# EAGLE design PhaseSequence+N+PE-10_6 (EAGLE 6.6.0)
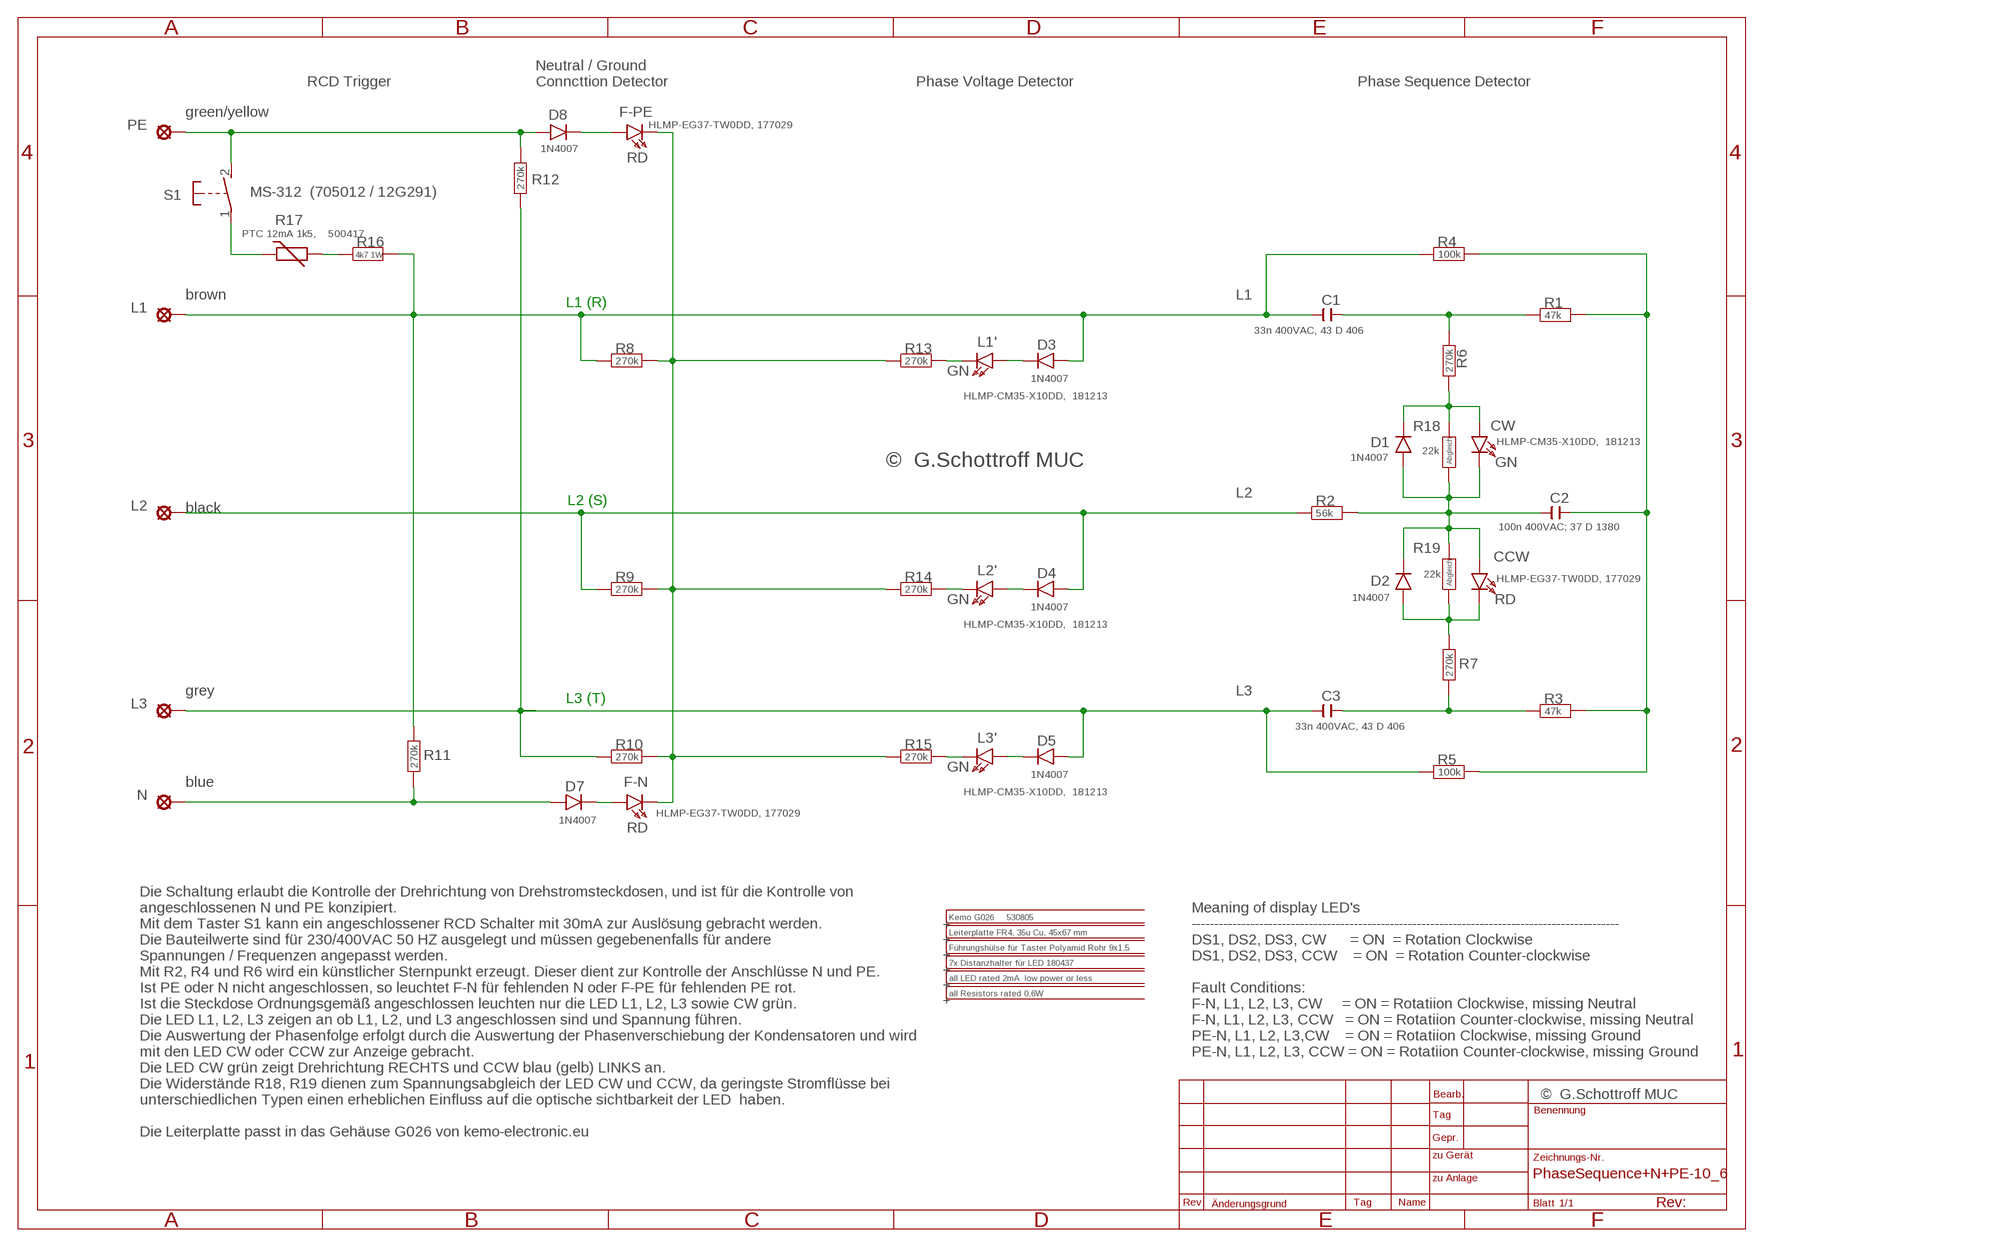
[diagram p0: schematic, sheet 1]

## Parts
C1  33n 400VAC, 43 D 406  C-EU150-064X183  [C150-064X183]
C2  100n 400VAC; 37 D 1380  C-EU150-084X183  [C150-084X183]
C3  33n 400VAC, 43 D 406  C-EU150-064X183  [C150-064X183]
CCW  HLMP-EG37-TW0DD, 177029  LED5MM  [LED5MM]
CW  HLMP-CM35-X10DD, 181213  LED5MM  [LED5MM]
D1  1N4007  1N4004  [DO41-10]
D2  1N4007  1N4004  [DO41-10]
D3  1N4007  1N4004  [DO41-10]
D4  1N4007  1N4004  [DO41-10]
D5  1N4007  1N4004  [DO41-10]
D7  1N4007  1N4004  [DO41-10]
D8  1N4007  1N4004  [DO41-10]
ENCLOSURE-1  Kemo G026 530805  KEMO-G025  [KEMO-G025]
F-N  HLMP-EG37-TW0DD, 177029  LED5MM  [LED5MM]
F-PE  HLMP-EG37-TW0DD, 177029  LED5MM  [LED5MM]
INFO1  Führungshülse für Taster Polyamid Rohr 9x1.5  INFO  [INFO]
INFO2  7x Distanzhalter für LED 180437  INFO  [INFO]
INFO3  all LED rated 2mA low power or less  INFO  [INFO]
INFO4  all Resistors rated 0,6W  INFO  [INFO]
L1  SE13  [SE13]
L1'  HLMP-CM35-X10DD, 181213  LED5MM  [LED5MM]
L2  SE13  [SE13]
L2'  HLMP-CM35-X10DD, 181213  LED5MM  [LED5MM]
L3  SE13  [SE13]
L3'  HLMP-CM35-X10DD, 181213  LED5MM  [LED5MM]
N  SE13  [SE13]
PCB  Leiterplatte FR4, 35u Cu, 45x67 mm  INFO  [INFO]
PE  SE13  [SE13]
R1  47k  R-EU_0207/10  [0207/10]
R2  56k  R-EU_0207/10  [0207/10]
R3  47k  R-EU_0207/10  [0207/10]
R4  100k  R-EU_0207/10  [0207/10]
R5  100k  R-EU_0207/10  [0207/10]
R6  270k  R-EU_0207/10  [0207/10]
R7  270k  R-EU_0207/10  [0207/10]
R8  270k  R-EU_0207/10  [0207/10]
R9  270k  R-EU_0207/10  [0207/10]
R10  270k  R-EU_0207/10  [0207/10]
R11  270k  R-EU_0207/10  [0207/10]
R12  270k  R-EU_0207/10  [0207/10]
R13  270k  R-EU_0207/10  [0207/10]
R14  270k  R-EU_0207/10  [0207/10]
R15  270k  R-EU_0207/10  [0207/10]
R16  4k7 1W  R-EU_0817/22  [P0817/22]
R17  PTC 12mA 1k5, 500417  THERMISTOR-5  [R-5]
R18  22k  R-EU_R1206  [1206]
R19  22k  R-EU_R1206  [1206]
S1  MS-312 (705012 / 12G291)  MS-312  [MS-312]

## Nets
L1: C1.2 D3.A L1.MP R4.1 R8.1 R11.2 R16.2
L2: D4.A L2.MP R2.1 R9.1
L3: C3.2 D5.A L3.MP R5.1 R10.1 R12.2
N$1: C3.1 R3.1 R7.1
N$2: C2.2 CCW.A CW.K(C) D1.A D2.C R2.2 R18.1 R19.2
N$3: C1.1 R1.1 R6.1
N$4: C2.1 R1.2 R3.2 R4.2 R5.2
N$5: CCW.K(C) D2.A R7.2 R19.1
N$6: CW.A D1.C R6.2 R18.2
N$7: F-N.K(C) F-PE.K(C) R8.2 R9.2 R10.2 R13.1 R14.1 R15.1
N$8: D7.A N.MP R11.1
N$9: L1'.K(C) R13.2
N$10: L2'.K(C) R14.2
N$11: D7.C F-N.A
N$12: D8.A PE.MP R12.1 S1.2(S)
N$13: D8.C F-PE.A
N$14: L3'.K(C) R15.2
N$15: R17.1 S1.1(P)
N$16: D3.C L1'.A
N$17: R16.1 R17.2
N$18: D4.C L2'.A
N$19: D5.C L3'.A

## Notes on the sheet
- RCD Trigger
- Neutral / Ground 
  Conncttion Detector
- Phase Voltage Detector | Phase Sequence Detector
- green/yellow
- RD
- brown
- L1 (R)
- GN
- Abgleich
- ©  G.Schottroff MUC | GN
- L2 (S)
- black
- Abgleich
- GN | RD
- grey
- L3 (T)
- GN
- blue
- RD
- Meaning of display LED's
  -----------------------------------------------------------------------------------------------
  DS1, DS2, DS3, CW      = ON  = Rotation Clockwise
  DS1, DS2, DS3, CCW    = ON  = Rotation Counter-clockwise
  
  Fault Conditions:
  F-N, L1, L2, L3, CW     = ON = Rotatiion Clockwise, missing Neutral
  F-N, L1, L2, L3, CCW   = ON = Rotatiion Counter-clockwise, missing Neutral
  PE-N, L1, L2, L3,CW    = ON = Rotatiion Clockwise, missing Ground
  PE-N, L1, L2, L3, CCW = ON = Rotatiion Counter-clockwise, missing Ground
- ©  G.Schottroff MUC
- Die Schaltung erlaubt die Kontrolle der Drehrichtung von Drehstromsteckdosen, und ist für die Kontrolle von 
  angeschlossenen N und PE konzipiert. 
  Mit dem Taster S1 kann ein angeschlossener RCD Schalter mit 30mA zur Auslösung gebracht werden.
  Die Bauteilwerte sind für 230/400VAC 50 HZ ausgelegt und müssen gegebenenfalls für andere 
  Spannungen / Frequenzen angepasst werden.
  Mit R2, R4 und R6 wird ein künstlicher Sternpunkt erzeugt. Dieser dient zur Kontrolle der Anschlüsse N und PE. 
  Ist PE oder N nicht angeschlossen, so leuchtet F-N für fehlenden N oder F-PE für fehlenden PE rot.
  Ist die Steckdose Ordnungsgemäß angeschlossen leuchten nur die LED L1, L2, L3 sowie CW grün.
  Die LED L1, L2, L3 zeigen an ob L1, L2, und L3 angeschlossen sind und Spannung führen.
  Die Auswertung der Phasenfolge erfolgt durch die Auswertung der Phasenverschiebung der Kondensatoren und wird 
  mit den LED CW oder CCW zur Anzeige gebracht.
  Die LED CW grün zeigt Drehrichtung RECHTS und CCW blau (gelb) LINKS an.
  Die Widerstände R18, R19 dienen zum Spannungsabgleich der LED CW und CCW, da geringste Stromflüsse bei 
  unterschiedlichen Typen einen erheblichen Einfluss auf die optische sichtbarkeit der LED  haben.
  
  Die Leiterplatte passt in das Gehäuse G026 von kemo-electronic.eu

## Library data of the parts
C1-C3 = rcl:C-EU: CAPACITOR, European symbol
CCW CW F-N F-PE L1' L2' L3' = led:LED: LED
D1-D5 D7 D8 = diode:1N4004: DIODE
ENCLOSURE-1 = Enclosures-DIN-Rail+more:KEMO-G025
INFO1-INFO4 PCB = frames:INFO
L1-L3 N PE = solpad:SE13: SOLDER PAD
R1-R16 R18 R19 = rcl:R-EU_: RESISTOR, European symbol
R17 = varistor:THERMISTOR: THERMISTOR
S1 = switch-misc:MS-312

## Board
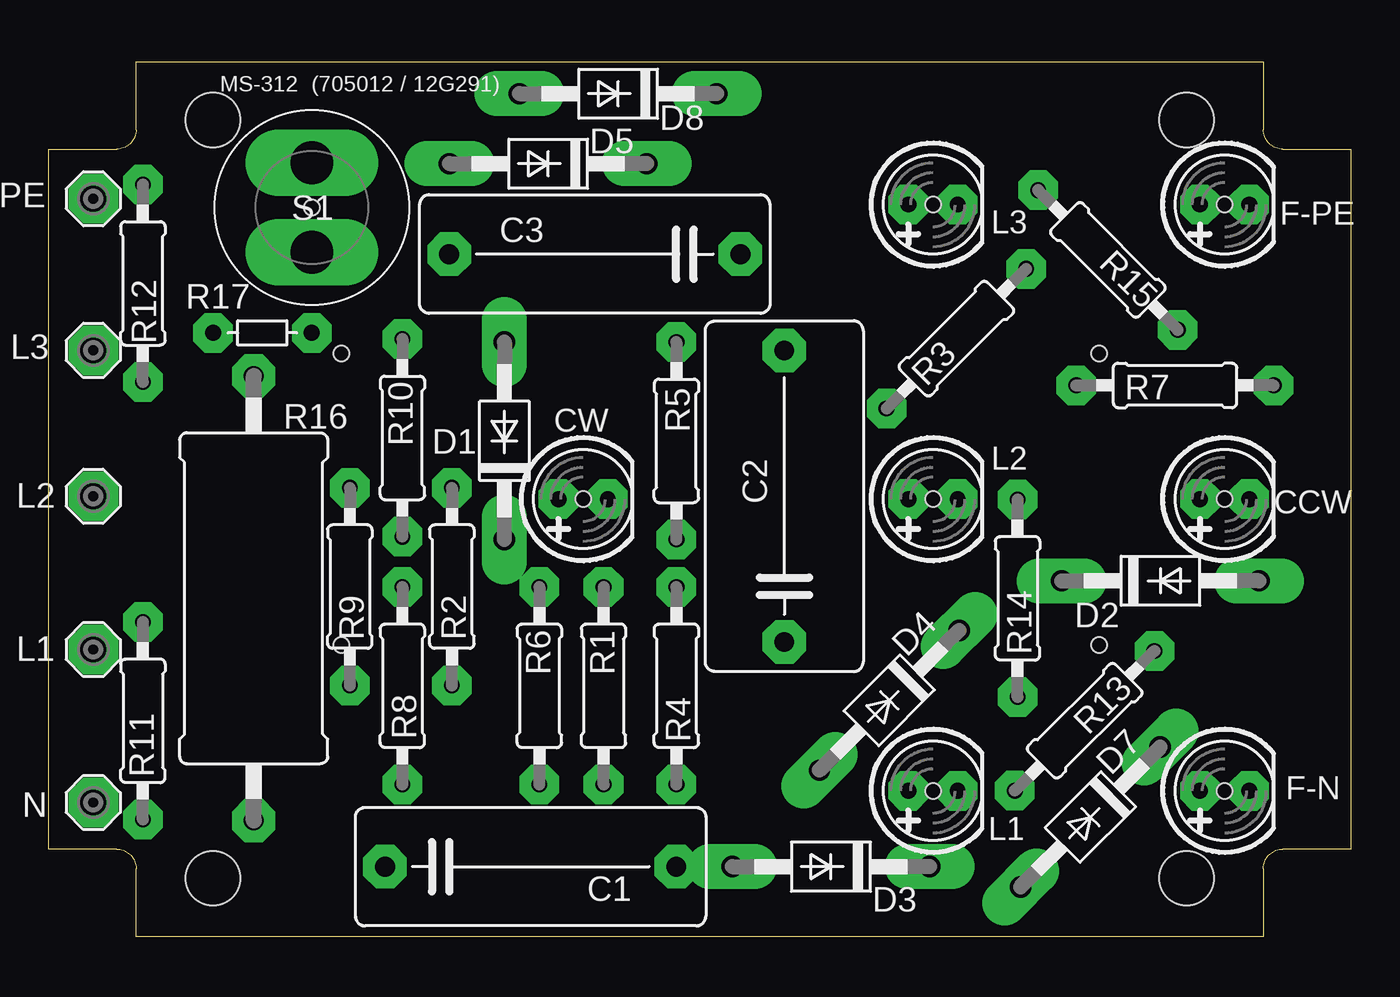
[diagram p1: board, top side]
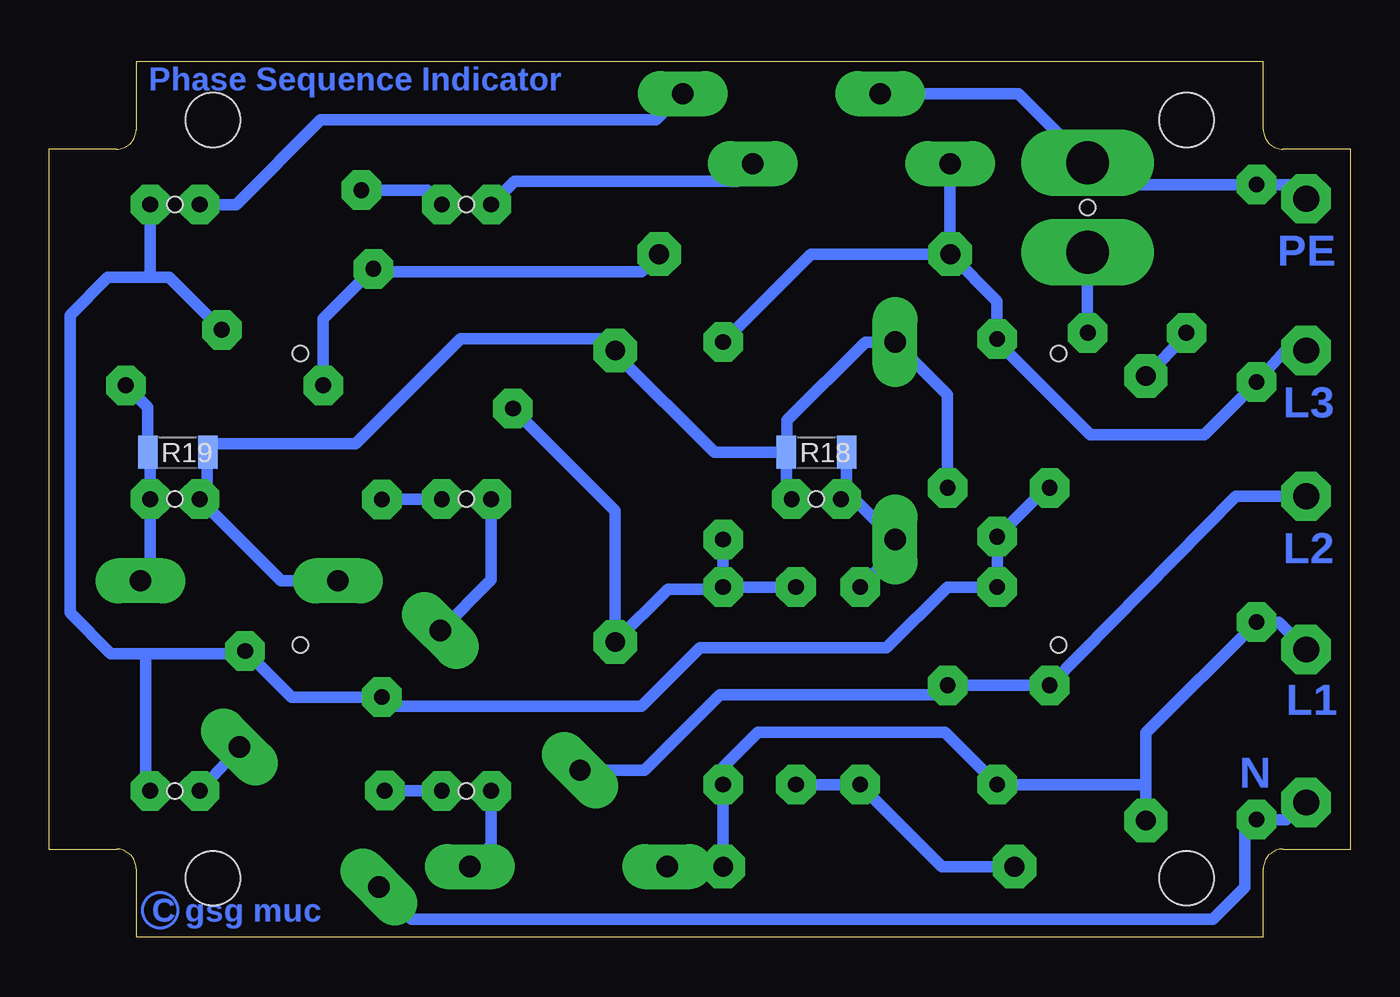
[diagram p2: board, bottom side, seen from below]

Size 67 x 45 mm. Coordinates in mm from the lower left corner, seen from the top.
Copper layers ((1*2)+(15*16)): Top 0.035mm / dielectric 0.7mm / Route2 0.035mm / dielectric 0.15mm / Route15 0.035mm / dielectric 0.7mm / Bottom 0.035mm
Design rules "default *": minimum track width 0.6mm, minimum drill 0.3mm, track to track 0.15mm, track to pad 0.15mm, pad to pad 0.15mm, via to via 0.15mm, smd to smd 2mil, copper to edge 20mil, drill to drill 7mil, minimum pad ring 24mil, minimum via ring 8mil, stop-mask expansion 0.05mm, vias tented up to drill 0.6mm, thermal gap 10mil
Holes 0.8 mm at 54.05,15 54.05,30 15.05,30 15.05,15 13.55,37.5 27.5,22.5 45.5,7.5 45.5,22.5 45.5,37.65 60.5,37.65 60.5,22.5 60.5,7.5

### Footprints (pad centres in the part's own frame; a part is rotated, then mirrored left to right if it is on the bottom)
C150-064X183 = drill 1.016 octagon: 1 -7.493,0; 2 7.493,0
C150-084X183 = drill 1.016 octagon: 1 -7.493,0; 2 7.493,0
LED5MM = drill 0.813 pad 1.676 octagon: A -1.27,0; K 1.27,0
DO41-10 = drill 1.1 long: A 5.08,0; C -5.08,0
KEMO-G025 = hole 2.8: -25.05,19.5; 25.05,19.5; 25.05,-19.5; -25.05,-19.5
SE13 = drill 1.321 pad 2.159 octagon: MP 0,0
0207/10 = drill 0.813 octagon: 1 -5.08,0; 2 5.08,0
P0817/22 = drill 1.016 octagon: 1 -11.43,0; 2 11.43,0
R-5 = drill 0.813 octagon: 1 -2.54,0; 2 2.54,0
1206 = smd 1 x 1.7: 1 -1.55,0; 2 1.55,0
MS-312 = drill 2.2 long: 1 -2.3,0; 2 2.3,0

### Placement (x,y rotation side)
C1  24.8,3.6 0 top
C2  37.85,22.65 90 top
C3  28.1,35.1 180 top
CCW  60.5,22.5 0 top
CW  27.5,22.5 0 top
D1  23.45,25.5 90 top
D2  57.2,18.3 0 top
D3  40.25,3.6 180 top
D4  43.25,12.15 225 top
D5  25.7,39.75 180 top
D7  53.6,6.15 225 top
D8  29.3,43.35 180 top
ENCLOSURE-1  33.5,22.5 0 top
F-N  60.5,7.5 0 top
F-PE  60.5,37.65 0 top
INFO1  not placed on the board
INFO2  not placed on the board
INFO3  not placed on the board
INFO4  not placed on the board
L1  2.3,14.77 0 top
L1'  45.5,7.5 0 top
L2  2.3,22.65 0 top
L2'  45.5,22.5 0 top
L3  2.3,30.15 0 top
L3'  45.5,37.65 0 top
N  2.3,6.9 0 top
PCB  5.9,-1.35 0 top
PE  2.3,37.95 0 top
R1  28.55,12.9 90 top
R2  20.75,18 90 top
R3  46.7,30.75 225 top
R4  32.3,12.9 90 top
R5  32.3,25.5 270 top
R6  25.25,12.9 90 top
R7  57.95,28.35 0 top
R8  18.2,12.9 90 top
R9  15.5,18 90 top
R10  18.2,25.65 270 top
R11  4.85,11.1 90 top
R12  4.85,33.6 270 top
R13  53.3,11.1 225 top
R14  49.85,17.4 90 top
R15  54.5,34.8 135 top
R16  10.55,17.4 270 top
R17  11,31.05 180 top
R18  27.5,24.9 0 bottom
R19  60.35,24.9 0 bottom
S1  13.55,37.5 90 top

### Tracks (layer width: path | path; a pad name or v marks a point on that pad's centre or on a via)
L1
  Bottom 0.6: L1.MP 3.71,16.18 R11.2 10.55,10.48 10.55,7.65 | D3.A C1.2 R4.1 32.3,8.7 30.5,10.5 20.88,10.5 R8.1 10.72,7.82 10.55,7.65 | R16.2 10.55,7.65
L2
  Bottom 0.6: L2.MP 5.92,22.65 R9.1 R2.1 20.75,12.9 21.2,12.45 32.45,12.45 36.35,8.55 D4.A
L3
  Bottom 0.6: L3.MP 3.37,30.15 R12.2 4.85,28.5 7.55,25.8 13.4,25.8 17.75,30.15 18.18,30.73 R10.1 18.21,32.69 C3.2 | C3.2 27.78,35.1 R5.1 | D5.A 20.62,35.11 C3.2
N$1
  Bottom 0.6: C3.1 36.5,34.2 47.02,34.2 50.15,34.2 R3.1 52.87,31.76 R7.1
N$2
  Bottom 0.6: R18.1 29,24.65 29,26.55 24.97,30.58 D1.A 20.75,27.88 R2.2 | R18.1 29.05,22.78 CW.K | C2.2 37.85,30 | 37.85,30 32.75,24.9 R18.1 | 37.85,30 38.6,30.75 45.8,30.75 51.2,25.35 58.65,25.35 R19.2 58.85,24.85 58.85,22.95 59.23,22.57 CCW.A 55.03,18.3 D2.C
N$3
  Bottom 0.6: R1.1 R6.1 21.03,3.6 C1.1
N$4
  Bottom 0.6: R1.2 R4.2 | R5.2 R4.2 | R4.2 32.6,17.85 32.61,17.86 35.12,17.86 C2.1 37.85,21.9 43.25,27.3 R3.2
N$5
  Bottom 0.6: D2.A 61.77,18.81 CCW.K 61.77,24.77 R19.1 61.9,27.22 R7.2
N$6
  Bottom 0.6: R18.2 25.95,22.78 CW.A 25.53,22.5 D1.C 23.45,19.78 R6.2
N$7
  Bottom 0.6: R9.2 15.65,23.12 R10.2 R8.2 20.77,17.98 23.9,14.85 33.5,14.85 36.5,11.85 49.4,11.85 R14.1 49.83,12.3 54.5,12.3 R13.1 57.03,14.55 61.85,14.55 | R15.1 58.11,31.21 60.8,33.9 62.15,33.9 | 62.15,33.9 63.95,33.9 65.9,31.95 65.9,16.65 63.8,14.55 61.85,14.55 | F-N.K 61.77,7.57 62,7.8 62,14.4 61.85,14.55 | F-PE.K 61.77,33.98 62.15,33.9
N$8
  Bottom 0.6: R11.1 3.33,6.02 N.MP | R11.1 4.83,5.87 5,6 4.87,6 R11.1 | D7.A 48.33,0.9 37.1,0.9 14.9,0.9 7.1,0.9 5.45,2.55 5.45,5.42 R11.1
N$9
  Bottom 0.6: L1'.K 49.27,7.5 R13.2
N$10
  Bottom 0.6: L2'.K 49.83,22.5 R14.2
N$11
  Bottom 0.6: D7.C 57.2,9.68 F-N.A
N$12
  Bottom 0.6: PE.MP 3.03,38.68 R12.1 12.43,38.68 S1.2 17.1,43.35 D8.A
N$13
  Bottom 0.6: D8.C 34.4,43.35 35.75,42 53,42 57.35,37.65 F-PE.A
N$14
  Bottom 0.6: R15.2 47.51,38.39 L3'.K
N$15
  Bottom 0.6: S1.1 R17.1
N$16
  Bottom 0.6: L1'.A 44.23,4.7 D3.C
N$17
  Bottom 0.6: R17.2 8.46,30.92 R16.1
N$18
  Bottom 0.6: L2'.A 44.23,18.35 D4.C
N$19
  Bottom 0.6: D5.C 30.65,39.75 31.55,38.85 43.03,38.85 L3'.A
(copper drawn outside any net)
  shapes: Bottom circle x9, Route15 circle x12

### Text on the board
Bottom: Phase Sequence Indicator | PE | L3 | L2 | L1 | N | C gsg muc
tNames: F-PE | L3 | CW | L2 | CCW | F-N | L1
Document: Rotation / CCW | Rotation / CW | Press Button for / 30mA RCD Test | = Line / OK | L1 L2 L3 | Fault_N Fault_PE | N=Missing PE= Missing
Reference: Polyamid / Rohr / 10x1,5 | > ON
